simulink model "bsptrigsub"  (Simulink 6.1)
settings: Solver=ode45  SolverMode=SingleTasking  StartTime=0.0  StopTime=10.0  FixedStep=0.01  RelTol=1e-3

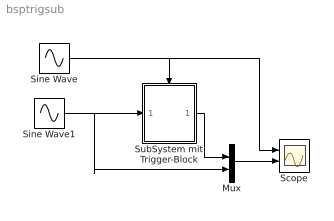
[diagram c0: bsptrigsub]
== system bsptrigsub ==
  Mux : Mux  Inputs=2
  Scope : Scope  NumInputPorts=2
  Sine Wave : Sin  Frequency=10  SampleTime=0
  Sine Wave1 : Sin  SampleTime=0
  SubSystem mit Trigger-Block : Subsystem
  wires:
  Sine Wave1/1 -> SubSystem mit Trigger-Block/1(In1), Mux/2
  SubSystem mit Trigger-Block/1(Out1) -> Mux/1
  Mux/1 -> Scope/2
  Sine Wave/1 -> SubSystem mit Trigger-Block/Trigger, Scope/1

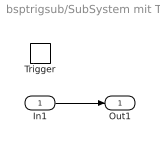
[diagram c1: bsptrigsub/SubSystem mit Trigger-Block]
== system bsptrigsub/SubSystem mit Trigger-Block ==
  In1 : Inport  Port=1  LatchInput=off
  Trigger : TriggerPort  TriggerType=either
  Out1 : Outport
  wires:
  In1/1 -> Out1/1
